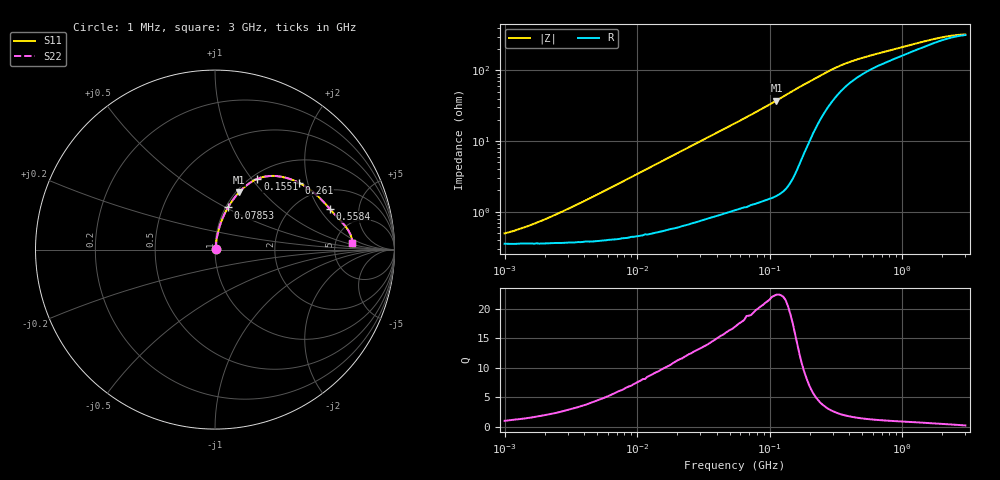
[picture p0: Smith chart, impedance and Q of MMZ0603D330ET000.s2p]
! S-Parameter Data Generated by TDK Corporation
! Copyright(C) 2025 TDK Corporation.
! All Rights Reserved.
! TDK P/N: MMZ0603D330ET000 (Chip Bead)
! Property: |Z|=33ohm at 100MHz
! Size(LxWxT): 0.6x0.3x0.3mm
! Model Type: s2p (Touchstone File Format Version 1.0)
! Frequency: DC=Yes Start=1MHz Stop=3000MHz 202points Log-sweep
! Model Generated on Feb. 6, 2025
! Terms and conditions regarding TDK Simulation Models:
! 1)This simulation model is being provided solely for informational
!  purposes. Please refer to the specifications of the products in
!  terms of detailed characteristics of such products.
! 2)In no event shall TDK Corporation of any of its subsidiaries be
!  liable for any loss or damage arising, directly or indirectly,
!  from any information contained in this simulation model, including,
!  but not limited to loss or damages arising from any inaccuracies,
!  omissions or errors in connection with such information.
! 3)Any and all copyrights on this simulation model are owned by
!  TDK Corporation.  Duplication or redistribution of this simulation
!  model without prior written permission from TDK Corporation
!  is prohibited.
! 4)This simulation model is subject to any modification or change
!  without any prior notice.
! 5)Neither TDK Corporation nor any of its subsidiaries shall make any
!  warranty, express or implied, including but not limited to the
!  correctness, implied warranties of merchantability and fitness for
!  a particular purpose with respect to this simulation models.
! 6)The use of this simulation model shall be deemed to have consented
!  to the terms and conditions hereof.
! Port Assignments:
!  1 ---@@@--- 2
! Applicable Conditions:
!  Temperature = 25 degC
!  DC Bias Current = 0 A
!  Small Signal Operation
# Hz S MA R 50
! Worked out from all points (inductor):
!   201 points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, 1 MHz to 3 GHz, reference 50 ohm
!   read as one part in series: L = 54.5 nH near 3.323 MHz
!   highest Q = 22.3 at 112.6 MHz (marker M1), where L = 52.9 nH
!   S11 on the Smith chart (normalised r, x): 1 MHz: 1.01, +0.01; 78.53 MHz: 1.03, +0.51; 155.1 MHz: 1.07, +1.07; 261 MHz: 1.52, +1.76; 558.4 MHz: 2.99, +2.51; 3 GHz: 7.33, +1.23
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1000000  0.004932 44.4  0.9965 -0.2  0.9965 -0.2  0.004932 44.4
1433740  0.006058 54.0  0.9965 -0.3  0.9965 -0.3  0.006058 54.0
1897447  0.007414 61.1  0.9964 -0.4  0.9964 -0.4  0.007414 61.1
2511129  0.009307 66.8  0.9964 -0.5  0.9964 -0.5  0.009307 66.8
3900413  0.01383 73.6  0.9962 -0.8  0.9962 -0.8  0.01383 73.6
1.461624e7  0.04893 81.2  0.9937 -2.8  0.9937 -2.8  0.04893 81.2
3.00453e7  0.09791 80.1  0.9879 -5.6  0.9879 -5.6  0.09791 80.1
5.477226e7  0.1739 76.6  0.9746 -10.0  0.9746 -10.0  0.1739 76.6
7.852918e7  0.2454 72.9  0.9571 -14.2  0.9571 -14.2  0.2454 72.9
1.125904e8  0.346 67.2  0.9229 -20.2  0.9229 -20.2  0.346 67.2
1.321429e8  0.4019 63.7  0.8972 -23.7  0.8972 -23.7  0.4019 63.7
1.550909e8  0.4597 59.1  0.8595 -27.3  0.8595 -27.3  0.4597 59.1
1.820241e8  0.5105 53.4  0.8073 -30.5  0.8073 -30.5  0.5105 53.4
2.136344e8  0.5535 46.9  0.7416 -33.0  0.7416 -33.0  0.5535 46.9
2.609752e8  0.5971 38.7  0.6516 -35.0  0.6516 -35.0  0.5971 38.7
3.188066e8  0.6291 31.6  0.5695 -35.4  0.5695 -35.4  0.6291 31.6
3.741707e8  0.6474 27.1  0.516 -34.8  0.516 -34.8  0.6474 27.1
5.583748e8  0.6791 19.4  0.4247 -32.1  0.4247 -32.1  0.6791 19.4
8.005644e8  0.7038 15.0  0.368 -29.6  0.368 -29.6  0.7038 15.0
1.931433e9  0.7585 6.5  0.261 -19.3  0.261 -19.3  0.7585 6.5
2.455801e9  0.765 4.4  0.2443 -13.8  0.2443 -13.8  0.765 4.4
3e9  0.766 2.6  0.2374 -8.4  0.2374 -8.4  0.766 2.6
